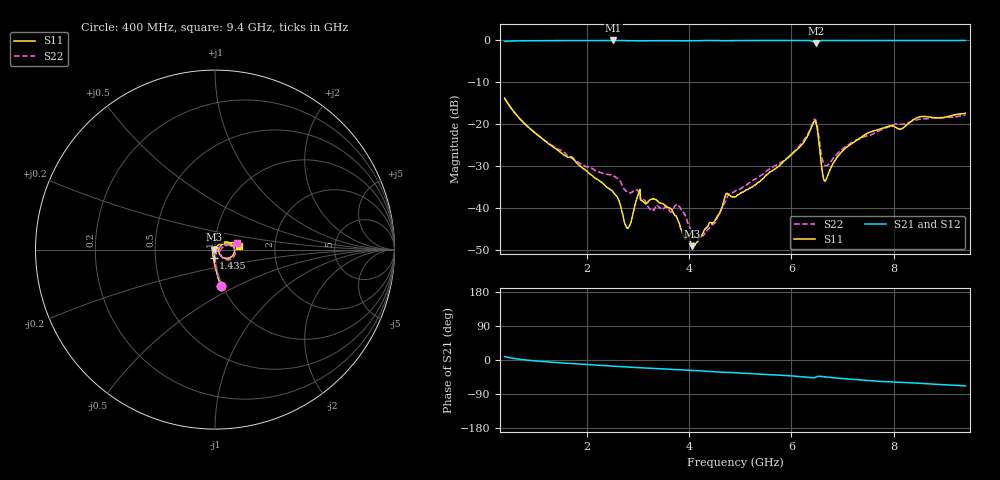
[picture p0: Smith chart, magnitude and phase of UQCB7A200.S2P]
!  Part Number  UQCB7A200  Mounting Orientation: Vertical
!  Description: RF capacitors
!  Application: Coupling, Bypass, Tuning, DC Block
!  Filters, Matching
# GHZ S DB R 50
! Freq  |S11|  S11 Ph  |S21|  S21 Ph  |S12|  S12 Ph  |S22|  S22 Ph
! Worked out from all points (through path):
!   801 points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, 400 MHz to 9.4 GHz, reference 50 ohm
!   highest |S21| = 0.00 dB at 2.526 GHz (marker M1); lowest = -0.6 dB at 6.486 GHz (marker M2)
!   group delay of S21, straight-line fit = 21.7 ps
!   lowest |S11| = -49.1 dB at 4.056 GHz (marker M3), VSWR 1.01, Z = 49.7 + j0.0329 ohm
!   |S11| at or under -10 dB: start of sweep to end of sweep
!   |S22| runs from -47.4 to -13.8 dB; largest |S21 - S12| = 0.0028
!   S11 on the Smith chart (normalised r, x): 400 MHz: 0.98, -0.41; 1.435 GHz: 0.98, -0.10; 9.4 GHz: 1.31, +0.05
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0.4  -13.78 -80.4  -0.21 9.1  -0.23 9.1  -13.77 -80.0
1.435  -26.17 -99.3  -0.04 -6.9  -0.06 -6.9  -25.93 -88.7
1.908  -30.32 -112.2  -0.04 -11.1  -0.06 -11.0  -29.57 -85.2
2.526  -36.25 -171.0  0.00 -16.1  -0.01 -16.1  -32.32 -74.1
2.796  -44.83 120.3  -0.05 -18.6  -0.06 -18.6  -36.11 -58.5
2.999  -37.17 115.0  -0.08 -20.0  -0.09 -20.0  -35.74 -31.0
3.246  -37.98 -87.7  -0.09 -21.6  -0.10 -21.6  -40.26 -94.6
3.404  -38.53 -101.6  -0.06 -22.8  -0.07 -22.7  -39.64 -92.4
3.798  -43.28 -146.4  -0.07 -25.9  -0.08 -25.8  -39.48 -129.8
4.056  -49.12 174.6  -0.08 -27.5  -0.09 -27.4  -45.82 153.7
4.293  -45.43 129.6  -0.03 -29.1  -0.04 -29.0  -46.44 77.8
4.563  -41.88 97.1  -0.02 -31.6  -0.03 -31.5  -42.09 60.4
4.731  -36.53 81.4  -0.08 -32.5  -0.09 -32.4  -37.76 53.4
4.9  -37.34 63.8  -0.03 -33.6  -0.04 -33.5  -35.96 36.8
5.958  -27.72 50.5  -0.01 -41.4  -0.01 -41.3  -27.76 29.5
6.408  -20.24 19.3  -0.19 -47.0  -0.19 -46.9  -19.92 9.5
6.486  -19.85 -21.3  -0.60 -44.7  -0.60 -44.6  -19.29 -26.4
6.61  -31.73 -33.1  -0.01 -43.7  -0.01 -43.6  -28.51 -35.9
6.666  -33.53 0.6  -0.01 -44.7  -0.01 -44.5  -29.92 -15.8
7.071  -25.58 34.9  -0.01 -49.7  -0.01 -49.5  -25.27 20.0
7.904  -20.46 18.6  -0.01 -57.5  -0.01 -57.4  -20.65 19.2
9.4  -17.39 8.1  -0.01 -68.2  -0.01 -68.0  -17.80 17.7
